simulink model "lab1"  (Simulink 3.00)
settings: Solver=ode1  SolverMode=SingleTasking  StartTime=0.0  StopTime=11  RelTol=1e-3  AbsTol=1e-6
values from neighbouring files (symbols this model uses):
  h = 0.01    [design.m]    (also in initfra.m; initlab1.m; tst.m)
  refseq = [0 1 1.001 2 2.001 3 3.001 4;            0 0 1     1 0     0 -1    -1]    [initfra.m]    (also in initlab1.m)
  Td = Sd    [design.m]    (also in makec2d.m; tst.m)
undefined symbols (not defined in the file or in its folder): Affd, Bffd, Rd
libraries: lab_lib x1, simulink3 x1

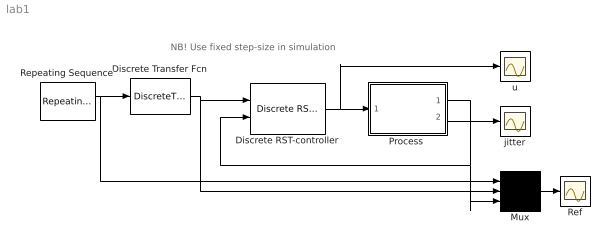
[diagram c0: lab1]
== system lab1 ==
  note: NB! Use fixed step-size in simulation
  Discrete Transfer Fcn : DiscreteTransferFcn  Numerator=Bffd  Denominator=Affd  SampleTime=h
  Discrete RST-controller : lab_lib/Discrete RST-controller  R=Rd  S=Sd  T=Td  h=h
  Mux : Mux  Inputs=3
  "Process " : Subsystem  mask(SISO Process){AOno=0, AIno=0, h=h}
      mask prompts: AOno "AO connection"; AIno "AI connection"; h "Sample Period"
      mask help: Process communication block. For use with Linux on PC with I/O.
  Ref : Scope
  Repeating Sequence : simulink3/Sources/Repeating Sequence  rep_seq_t=refseq(1,:)  rep_seq_y=refseq(2,:)
  jitter : Scope
  u : Scope
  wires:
  Discrete RST-controller/1 -> "Process "/1(AO), u/1
  Discrete Transfer Fcn/1 -> Discrete RST-controller/1, Mux/2
  "Process "/2(jitter) -> jitter/1
  Repeating Sequence/1 -> Discrete Transfer Fcn/1, Mux/1
  Mux/1 -> Ref/1
  "Process "/1(AI) -> Discrete RST-controller/2, Mux/3

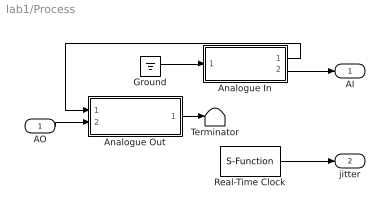
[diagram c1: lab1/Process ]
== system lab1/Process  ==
  AO : Inport  Port=1  PortWidth=-1  SampleTime=-1  DataType=auto
  Analogue In : Subsystem  mask(AnalogueIOBlock){h=h, AIno=AIno}
      mask prompts: h "Sample period"; AIno "Input port number"
      mask help: Analogue input block for use on PC running Linux.
  Analogue Out : Subsystem  mask(AnalogueIOBlock){h=h, AOno=AOno}
      mask prompts: h "Sample period"; AOno "Output port number"
      mask help: Analogue output block for use on PC running Linux
  Ground : Ground
  Real-Time Clock : S-Function  FunctionName=timer  Parameters=h  PortCounts=[]  SFunctionModules=''
  Terminator : Terminator
  AI : Outport  Port=1  InitialOutput=0
  jitter : Outport  Port=2
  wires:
  Ground/1 -> Analogue In/1(SortIn)
  Analogue In/2(Value) -> AI/1
  Real-Time Clock/1 -> jitter/1
  AO/1 -> Analogue Out/2(Value)
  Analogue In/1(SortOut) -> Analogue Out/1(SortIn)
  Analogue Out/1(SortOut) -> Terminator/1

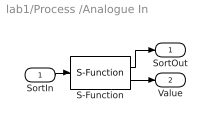
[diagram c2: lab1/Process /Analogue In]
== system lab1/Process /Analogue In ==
  SortIn : Inport  Port=1  PortWidth=-1  SampleTime=-1  DataType=auto
  S-Function : S-Function  FunctionName=analogin  Parameters=h AIno  PortCounts=[]  SFunctionModules=''
  SortOut : Outport  Port=1  InitialOutput=0
  Value : Outport  Port=2  InitialOutput=0
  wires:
  S-Function/2 -> Value/1
  SortIn/1 -> S-Function/1
  S-Function/1 -> SortOut/1

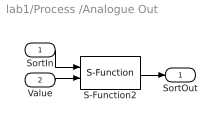
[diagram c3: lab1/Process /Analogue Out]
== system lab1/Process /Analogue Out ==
  SortIn : Inport  Port=1  PortWidth=-1  SampleTime=-1  DataType=auto
  Value : Inport  Port=2  PortWidth=-1  SampleTime=-1  DataType=auto
  S-Function2 : S-Function  FunctionName=analogout  Parameters=h AOno  PortCounts=[]  SFunctionModules=''
  SortOut : Outport  Port=1  InitialOutput=0
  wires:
  Value/1 -> S-Function2/2
  S-Function2/1 -> SortOut/1
  SortIn/1 -> S-Function2/1
